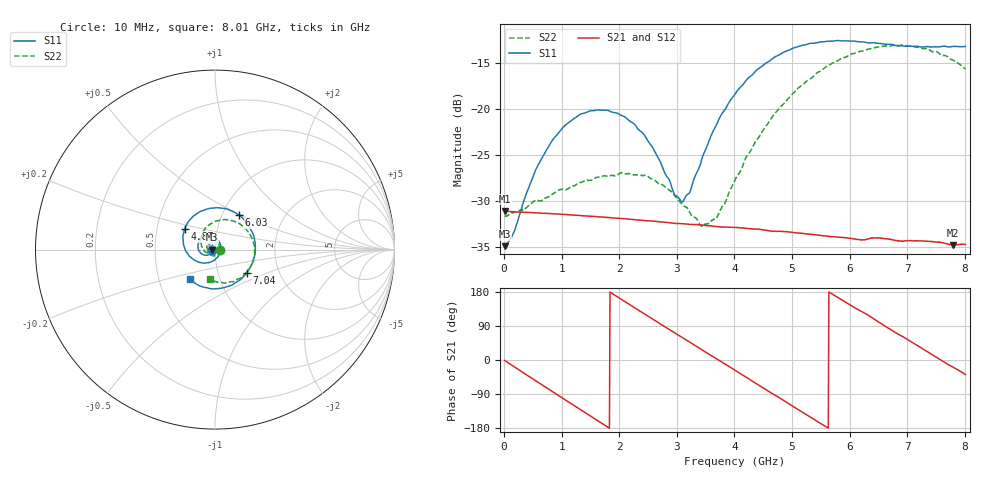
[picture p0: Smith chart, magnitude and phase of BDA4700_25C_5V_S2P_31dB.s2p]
!Agilent Technologies,E5071B,MY42404982,A.09.10
!Date: Mon Oct 20 13:42:14 2025
!Data & Calibration Information:
!Freq	S11:SOLT2(ON)	S21:SOLT2(ON)	S12:SOLT2(ON)	S22:SOLT2(ON)
# Hz S RI R 50
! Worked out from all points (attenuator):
!   801 points, 10 MHz to 8.01 GHz, reference 50 ohm
!   highest |S21| = -31.05 dB at 20 MHz (marker M1); lowest = -34.8 dB at 7.79 GHz (marker M2)
!   lowest |S11| = -34.9 dB at 10 MHz (marker M3), VSWR 1.04, Z = 48.2 - j0.0939 ohm
!   |S11| at or under -10 dB: start of sweep to end of sweep
!   |S22| runs from -32.7 to -13.0 dB; largest |S21 - S12| = 0.00024
!   S11 on the Smith chart (normalised r, x): 10 MHz: 0.96, -0.00; 4.87 GHz: 0.69, +0.17; 6.03 GHz: 1.21, +0.49; 7.04 GHz: 1.37, -0.37; 8.01 GHz: 0.72, -0.25
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1e7  -0.018 -0.000973  0.028 -0.000605  0.028 -0.000601  0.0262 -0.000825
2e7  -0.0184 -0.00162  0.028 -0.00104  0.028 -0.00114  0.0262 -0.00109
1.6e8  -0.0189 -0.00945  0.0267 -0.00774  0.0267 -0.00775  0.0264 -0.00756
5.3e8  -0.0352 -0.0285  0.0166 -0.0218  0.0166 -0.0219  0.0162 -0.0275
7.7e8  -0.0541 -0.0314  0.00638 -0.0264  0.00634 -0.0264  0.00107 -0.0335
1.35e9  -0.0945 0.00505  -0.0181 -0.0192  -0.0181 -0.0193  -0.036 -0.0178
2.09e9  -0.0518 0.075  -0.0231 0.0107  -0.0231 0.0108  -0.0293 0.0339
2.68e9  0.019 0.0507  -0.00361 0.0243  -0.00363 0.0243  0.0126 0.0375
2.96e9  0.0319 0.0127  0.00745 0.0228  0.00745 0.0228  0.0254 0.0229
3.11e9  0.0301 -0.0101  0.0127 0.0203  0.0127 0.0203  0.028 0.0109
3.41e9  0.00521 -0.0501  0.0205 0.0117  0.0205 0.0116  0.0205 -0.0113
3.54e9  -0.0125 -0.0633  0.0224 0.00685  0.0224 0.00686  0.0131 -0.0201
3.7e9  -0.0409 -0.073  0.0231 0.000845  0.0231 0.000792  -0.000547 -0.0261
4.01e9  -0.1012 -0.0655  0.0203 -0.0104  0.0203 -0.0104  -0.0321 -0.0258
4.87e9  -0.1694 0.1148  -0.00682 -0.0206  -0.00677 -0.0206  -0.0744 0.0785
5.35e9  -0.0758 0.2148  -0.0187 -0.00929  -0.0187 -0.00934  -0.0155 0.1477
6.03e9  0.1354 0.191  -0.016 0.0119  -0.016 0.0119  0.1372 0.1445
6.68e9  0.2246 -0.00899  0.00235 0.0196  0.0024 0.0197  0.2198 0.00131
7.04e9  0.1774 -0.1292  0.0122 0.015  0.0123 0.015  0.1979 -0.0957
7.43e9  0.0601 -0.2089  0.0186 0.00469  0.0186 0.00467  0.1198 -0.1675
7.79e9  -0.0728 -0.2064  0.0173 -0.00577  0.0174 -0.00585  0.0236 -0.183
8.01e9  -0.1417 -0.1666  0.0145 -0.0114  0.0146 -0.0114  -0.0299 -0.1625
